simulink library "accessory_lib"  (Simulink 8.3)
settings: Solver=ode45  StartTime=0.0  StopTime=10.0  RelTol=1e-3
undefined symbols (not defined in the file or in its folder): accessory
libraries: audit_lib x4, accessory_lib x4, general_lib x2

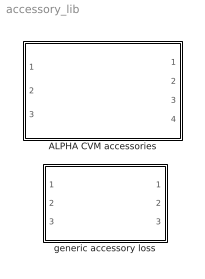
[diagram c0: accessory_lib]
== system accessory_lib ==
  ALPHA CVM accessories : Subsystem  VariantControl=variants_electric_ALPHA
  generic accessory loss : Subsystem

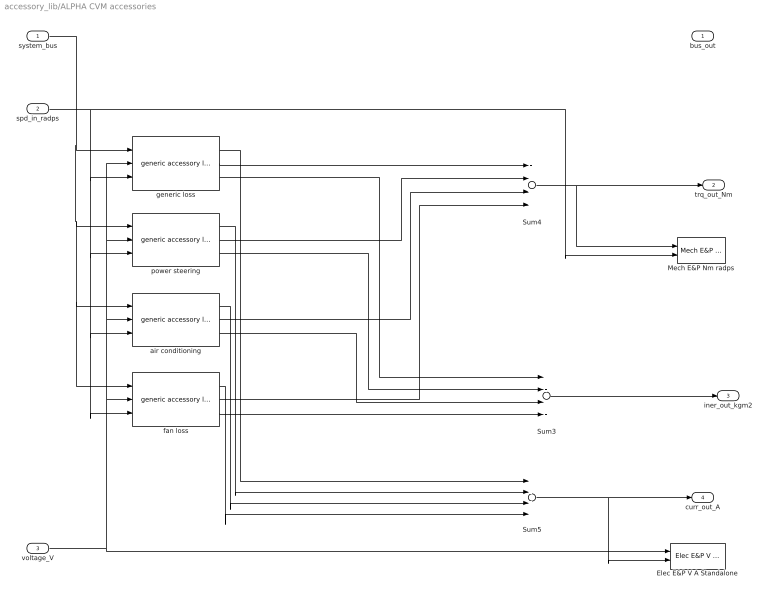
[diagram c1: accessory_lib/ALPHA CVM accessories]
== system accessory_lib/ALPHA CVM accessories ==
  system_bus : Inport
  spd_in_radps : Inport  Port=2
  voltage_V : Inport  Port=3
  Elec E&P V A Standalone : audit_lib/Elec E&P V A Standalone  base_name=accessories.total  VerboseSignal=REVS.verbose
  Mech E&P Nm radps : audit_lib/Mech E&P Nm radps0  base_name=accessories.total  VerboseSignal=REVS.verbose
  Sum3 : Sum  Inputs=++++
  Sum4 : Sum  Inputs=++++
  Sum5 : Sum  Inputs=++++
  air conditioning : accessory_lib/generic accessory loss  AuditBaseName=accessories.air_conditioner  accessory=accessories.air_conditioner
  fan loss : accessory_lib/generic accessory loss  AuditBaseName=accessories.fan  accessory=accessories.fan
  generic loss : accessory_lib/generic accessory loss  AuditBaseName=accessories.generic_loss  accessory=accessories.generic_loss
  power steering : accessory_lib/generic accessory loss  AuditBaseName=accessories.power_steering  accessory=accessories.power_steering
  bus_out : Outport
  trq_out_Nm : Outport  Port=2
  iner_out_kgm2 : Outport  Port=3
  curr_out_A : Outport  Port=4
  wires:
  generic loss/2 -> Sum4/1
  generic loss/3 -> Sum3/1
  Sum4/1 -> trq_out_Nm/1, Mech E&P Nm radps/1
  Sum3/1 -> iner_out_kgm2/1
  system_bus/1 -> fan loss/1, air conditioning/1, power steering/1, generic loss/1
  voltage_V/1 -> generic loss/2, power steering/2, air conditioning/2, fan loss/2, Elec E&P V A Standalone/1
  generic loss/1 -> Sum5/1
  power steering/1 -> Sum5/2
  air conditioning/1 -> Sum5/3
  fan loss/1 -> Sum5/4
  spd_in_radps/1 -> fan loss/3, air conditioning/3, power steering/3, generic loss/3, Mech E&P Nm radps/2
  power steering/2 -> Sum4/2
  air conditioning/2 -> Sum4/3
  fan loss/2 -> Sum4/4
  power steering/3 -> Sum3/2
  air conditioning/3 -> Sum3/3
  fan loss/3 -> Sum3/4
  Sum5/1 -> curr_out_A/1, Elec E&P V A Standalone/2

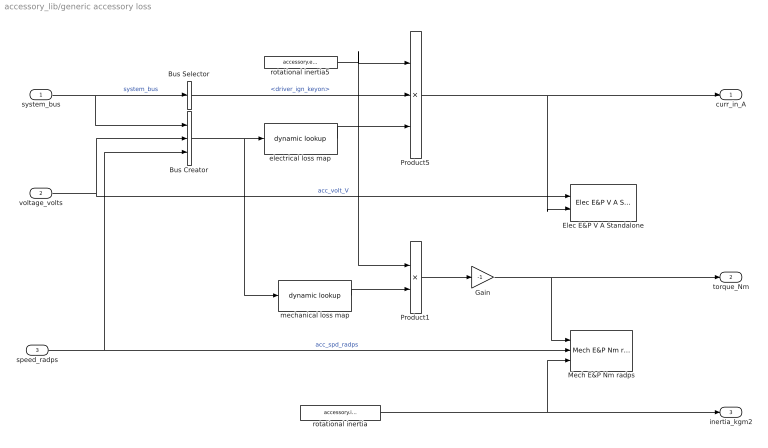
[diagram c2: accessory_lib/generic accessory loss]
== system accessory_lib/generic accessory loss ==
  system_bus : Inport
  voltage_volts : Inport  Port=2
  speed_radps : Inport  Port=3
  Bus Creator : BusCreator  Inputs=3
  Bus Selector : BusSelector  OutputSignals=driver.driver_ign_keyon
  Elec E&P V A Standalone : audit_lib/Elec E&P V A Standalone  base_name=constant_power_accessories  VerboseSignal=REVS.verbose
  Gain : Gain  Gain=-1
  Mech E&P Nm radps : audit_lib/Mech E&P Nm radps  base_name=constant_power_accessories  VerboseSignal=REVS.verbose
  Product1 : Product  Inputs=**
  Product5 : Product  Inputs=***
  electrical loss map : general_lib/dynamic lookup  LookupStructure=accessory.electrical_loss_map_A  InterpMethod=Linear  ExtrapMethod=Clip  DiagnosticForOutOfRangeInput=Warning  IndexSearchMethod=Linear search  BeginIndexSearchUsingPreviousIndexResult=on  SupportTunableTableSize=off  LookupStructureEval=|
      | LookupStructure =
      | 
      |      []
  mechanical loss map : general_lib/dynamic lookup  LookupStructure=accessory.mechanical_loss_map_Nm  InterpMethod=Linear  ExtrapMethod=Clip  DiagnosticForOutOfRangeInput=Warning  IndexSearchMethod=Linear search  BeginIndexSearchUsingPreviousIndexResult=on  SupportTunableTableSize=off  LookupStructureEval=|
      | LookupStructure =
      | 
      |      []
  rotational inertia : Constant  Value=accessory.inertia_kgm2
  rotational inertia5 : Constant  Value=accessory.enable
  curr_in_A : Outport
  torque_Nm : Outport  Port=2
  inertia_kgm2 : Outport  Port=3
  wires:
  system_bus/1 -> Bus Selector/1, Bus Creator/1  "system_bus"
  voltage_volts/1 -> Elec E&P V A Standalone/1, Bus Creator/2  "acc_volt_V"
  Product5/1 -> Elec E&P V A Standalone/2, curr_in_A/1
  Gain/1 -> Mech E&P Nm radps/1, torque_Nm/1
  rotational inertia/1 -> Mech E&P Nm radps/3, inertia_kgm2/1
  speed_radps/1 -> Mech E&P Nm radps/2, Bus Creator/3  "acc_spd_radps"
  electrical loss map/1 -> Product5/3
  rotational inertia5/1 -> Product1/1, Product5/1
  mechanical loss map/1 -> Product1/2
  Bus Selector/1 -> Product5/2  "<driver_ign_keyon>"
  Product1/1 -> Gain/1
  Bus Creator/1 -> mechanical loss map/1, electrical loss map/1
